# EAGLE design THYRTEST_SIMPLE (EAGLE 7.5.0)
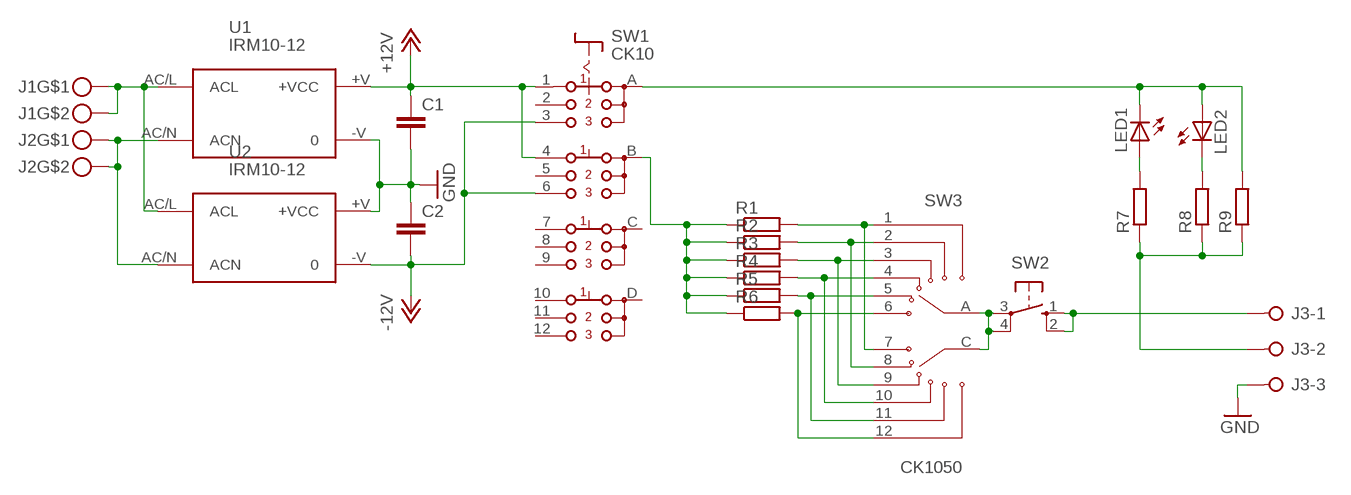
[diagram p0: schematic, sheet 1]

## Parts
C1  C-EUC1206  [C1206]
C2  C-EUC1206  [C1206]
J1  MKDSN1,5-2-5,08  [MKDSN1,5-2-5,08]
J2  MKDSN1,5-2-5,08  [MKDSN1,5-2-5,08]
J3  W237-3E  [W237-3E]
LED1  LED5MM  [LED5MM]
LED2  LED5MM  [LED5MM]
R1  R-EU_M1206  [M1206]
R2  R-EU_M1206  [M1206]
R3  R-EU_M1206  [M1206]
R4  R-EU_M1206  [M1206]
R5  R-EU_M1206  [M1206]
R6  R-EU_M1206  [M1206]
R7  R-EU_M1206  [M1206]
R8  R-EU_M1206  [M1206]
R9  R-EU_R2512  [R2512]
SW1  CK10  [CK10]
SW2  40-XX  [B3F-40XX]
SW3  CK1050  [SW_CK1050]
U1  IRM10-12  [IRM10-12]
U2  IRM10-12  [IRM10-12]

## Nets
+12V: C1.1 SW1.1(A1) SW1.4(B1) U1.+V(+VCC)
-12V: C2.2 SW1.3(A3) SW1.6(B3) U2.-V
GND: C1.2 C2.1 J3.3 U1.-V U2.+V(+VCC)
N$1: J2.1 J2.2 U1.AC/N(ACN) U2.AC/N(ACN)
N$2: R1.1 R2.1 R3.1 R4.1 R5.1 R6.1 SW1.B
N$3: R1.2 SW3.1 SW3.7
N$4: J1.1 J1.2 U1.AC/L(ACL) U2.AC/L(ACL)
N$5: R2.2 SW3.2 SW3.8
N$6: R3.2 SW3.3 SW3.9
N$7: R4.2 SW3.4 SW3.10
N$8: R5.2 SW3.5 SW3.11
N$9: R6.2 SW3.6 SW3.12
N$10: J3.1 SW2.1(S) SW2.2(S1)
N$11: LED1.A R7.2
N$12: LED1.K(C) LED2.A R9.2 SW1.A
N$13: LED2.K(C) R8.2
N$15: SW2.3(P) SW2.4(P1) SW3.A SW3.C
N$17: J3.2 R7.1 R8.1 R9.1
Unconnected: SW1.2(A2) SW1.5(B2) SW1.7(C1) SW1.8(C2) SW1.9(C3) SW1.10(D1) SW1.11(D2) SW1.12(D3) SW1.C SW1.D

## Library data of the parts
C1 C2 = rcl:C-EU: CAPACITOR, European symbol
J1 J2 = con-phoenix-508:MKDSN1,5-2-5,08
J3 = con-wago-508:W237-3E: WAGO SREW CLAMP; OC_FARNELL: unknown; OC_NEWARK: unknown
LED1 LED2 = led:LED: LED
R1-R9 = rcl:R-EU_: RESISTOR, European symbol
SW1 = switch:CK10: ROTARY SWITCH C&K
SW2 = switch-omron:40-XX: OMRON SWITCH; MF: OMRON COMPONENTS USA; MPN: B3F-4000; OC_FARNELL: 176434; OC_NEWARK: 36K3105
SW3 = CK1050:CK1050: Check availability; AVAILABILITY: In Stock; CHECK_PRICES: https://www.snapeda.com/parts/CK1050/Lorlin/view-part/?ref=eda; DESCRIPTION: Rotary wafer switch,metric,BBM,2P 6way | Lorlin CK1050; MF: Lorlin; MP: CK1050; PACKAGE: None; PRICE: None; SNAPEDA_LINK: https://www.snapeda.com/parts/CK1050/Lorlin/view-part/?ref=snap
U1 U2 = acdc:IRM10-12

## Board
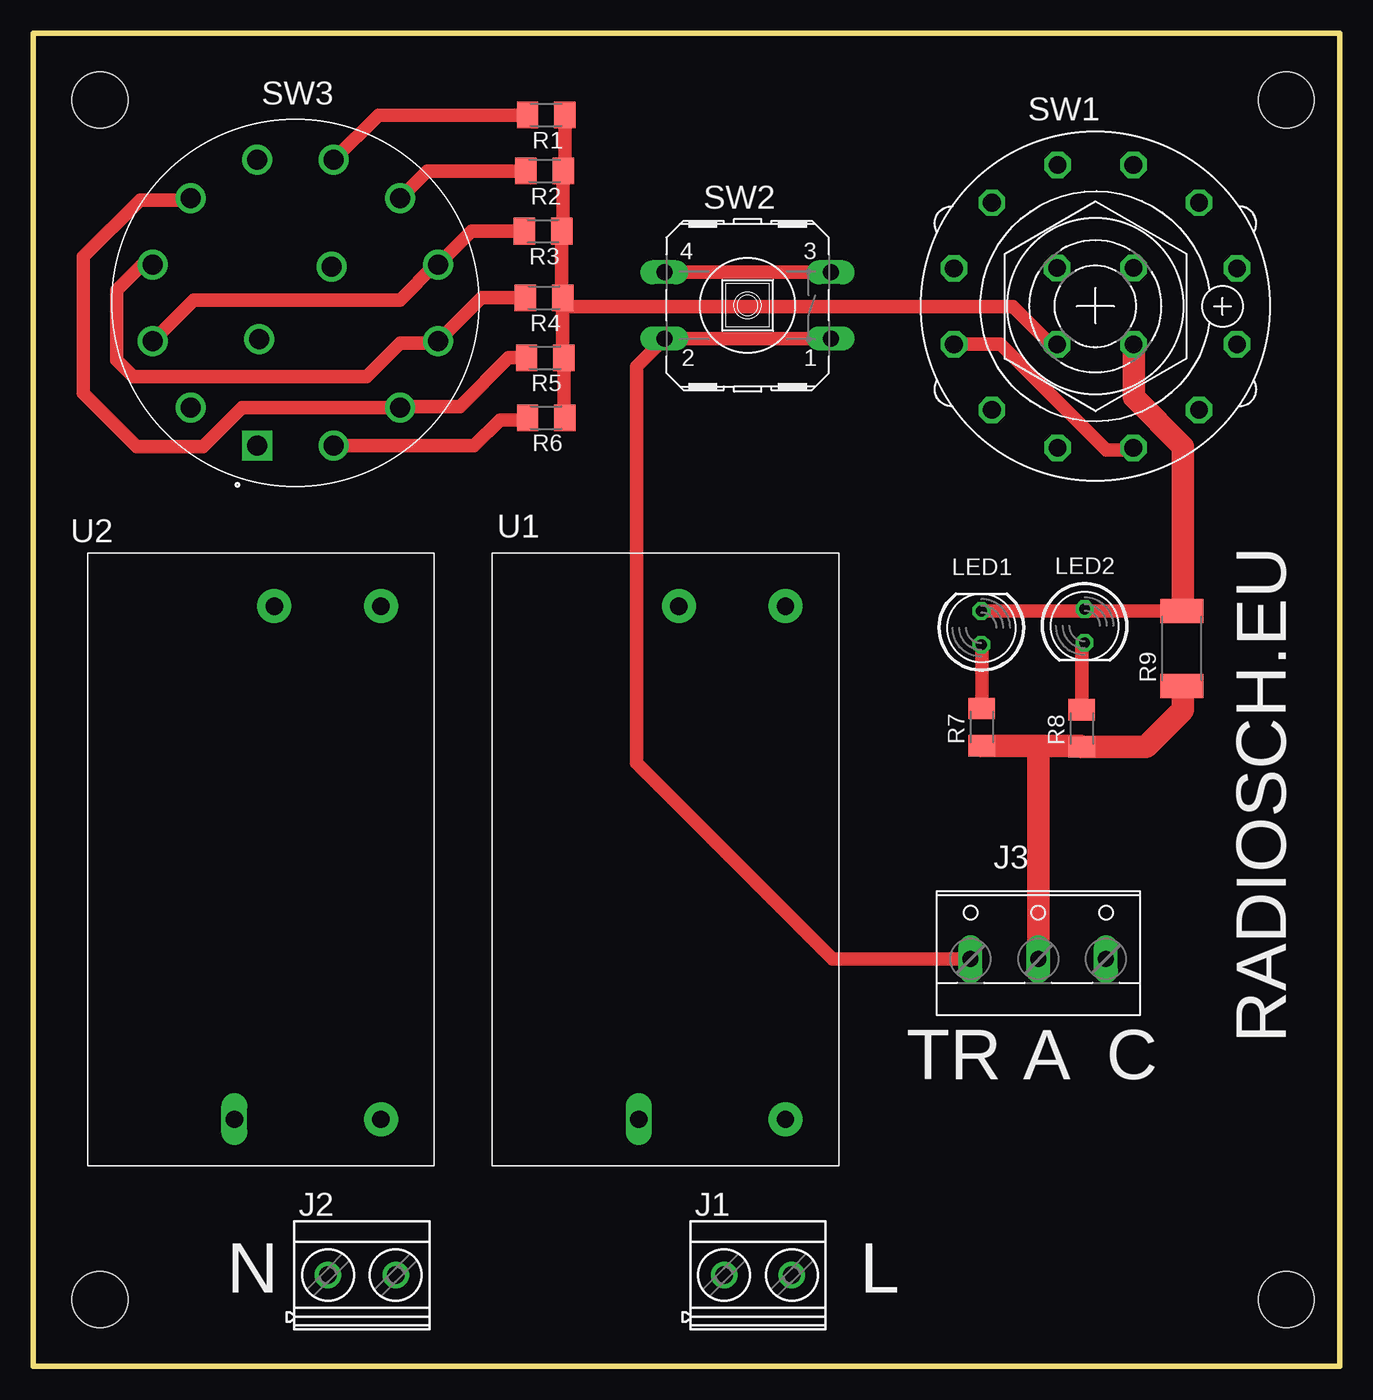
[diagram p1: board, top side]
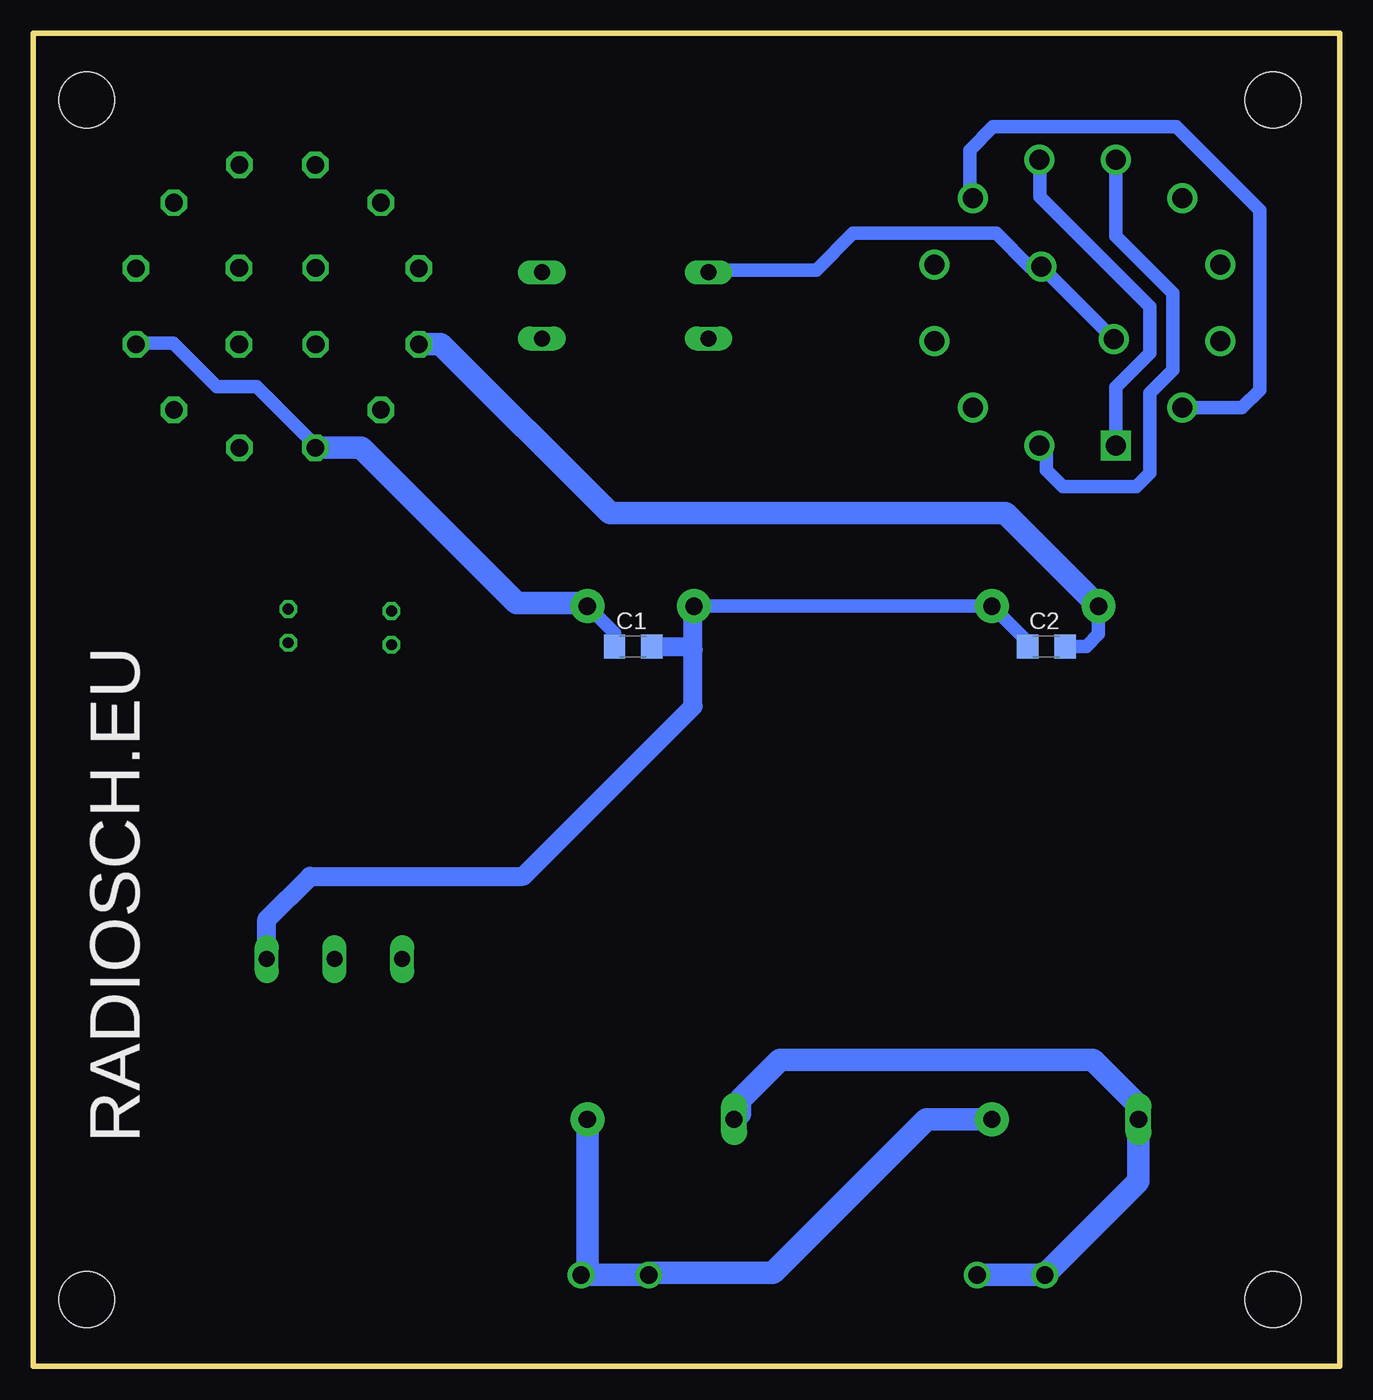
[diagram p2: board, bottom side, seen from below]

Size 98 x 100 mm. Coordinates in mm from the lower left corner, seen from the top.
Outline: 0,0 98,0 98,100 0,100 0,0
Copper layers (1*16): Top 0.035mm / dielectric 1.5mm / Bottom 0.035mm
Design rules "default": minimum track width 10mil, minimum drill 24mil, track to track 8mil, track to pad 8mil, pad to pad 8mil, via to via 8mil, smd to smd 8mil, copper to edge 40mil, drill to drill 8mil, minimum pad ring 10mil, minimum via ring 8mil, stop-mask expansion 4mil, vias tented up to drill 0mil, thermal gap 10mil
Holes 4.2 mm at 5,5 94,5 5,95 94,95

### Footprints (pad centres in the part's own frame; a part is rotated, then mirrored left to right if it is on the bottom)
C1206 = smd 1.6 x 1.8: 1 -1.4,0; 2 1.4,0
MKDSN1,5-2-5,08 = drill 1.3 pad 2: 1 -2.561,0.025; 2 2.519,0.025
W237-3E = drill 1.194 long: 1 -5.08,-0.635; 2 0,-0.635; 3 5.08,-0.635
LED5MM = drill 0.813 octagon: A -1.27,0; K 1.27,0
M1206 = smd 1.6 x 2: 1 -1.4,0; 2 1.4,0
R2512 = smd 1.8 x 3.2: 1 -2.8,0; 2 2.8,0
CK10 = drill 1.321 octagon: 1 -2.845,-10.617; 2 -7.772,-7.772; 3 -10.617,-2.845; 4 -10.617,2.845; 5 -7.772,7.772; 6 -2.845,10.617; 7 2.845,10.617; 8 7.772,7.772; 9 10.617,2.845; 10 10.617,-2.845; 11 7.772,-7.772; 12 2.845,-10.617; A -2.87,-2.87; B -2.87,2.87; C 2.87,2.87; D 2.87,-2.87
B3F-40XX = drill 1.194 long: 1 -6.248,2.489; 2 6.248,2.489; 3 -6.248,-2.489; 4 6.248,-2.489
SW_CK1050 = drill 1.5 square: 1 -2.873,-10.722 | drill 1.5: 2 -7.849,-7.849; 3 -10.722,-2.873; 4 -10.722,2.873; 5 -7.849,7.849; 6 -2.873,10.722; 7 2.873,10.722; 8 7.849,7.849; 9 10.722,2.873; 10 10.722,-2.873; 11 7.849,-7.849; 12 2.873,-10.722; A -2.722,-2.722; C 2.722,2.722
IRM10-12 = drill 1.3 pad 2.54: +V 38.5,0; -V 38.5,8; AC/L 0,0 | drill 1.3 long: AC/N 0,11

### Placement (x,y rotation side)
C1  53,54 0 bottom
C2  22,54 0 bottom
J1  54.39,6.82 0 top
J2  24.67,6.82 0 top
J3  75.4,31.18 0 top
LED1  71.13,55.39 90 top
LED2  78.87,55.54 270 top
R1  38.48,93.87 180 top
R2  38.36,89.67 180 top
R3  38.24,85.16 180 top
R4  38.32,80.16 180 top
R5  38.4,75.66 180 top
R6  38.48,71.16 180 top
R7  71.16,47.94 90 top
R8  78.66,47.86 90 top
R9  86.17,53.84 90 top
SW1  79.69,79.52 90 top
SW2  53.59,79.59 180 top
SW3  19.66,79.78 0 top
U1  56.43,18.52 90 top
U2  26.08,18.52 90 top

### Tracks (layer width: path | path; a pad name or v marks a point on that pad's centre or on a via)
+12V
  Bottom 1.016: SW1.4 76.84,69.09 81.25,73.5 84.25,73.5 87.5,76.75 90.23,76.75 SW1.1 | C1.1 54.4,54.99 U1.+V
  Bottom 1.676: SW1.4 73.4,68.9 61.75,57.25 56.66,57.25 U1.+V
-12V
  Top 1.016: SW1.6 72.58,76.67 80.5,68.75 82.38,68.75 SW1.3
  Bottom 1.016: U2.-V 18.08,54.92 19,54 C2.2
  Bottom 1.676: SW1.6 67.42,76.67 54.75,64 25.06,64 U2.-V
GND
  Bottom 1.016: 48.75,55 48.75,56.7 U1.-V U2.+V 23.4,54.34 C2.1
  Bottom 1.422: J3.3 80.48,33.52 77.25,36.75 61.25,36.75 48.5,49.5 48.5,53.75 | 48.5,53.75 48.5,56.95 U1.-V | C1.2 48.75,54 48.5,53.75
N$1
  Bottom 1.676: U1.AC/N 45,18.95 45,20 42,23 18.5,23 15.08,19.58 U2.AC/N 15.08,13.87 J2.1 J2.2
N$2
  Top 1.016: R1.1 39.88,89.79 R2.1 39.76,85.28 R3.1 39.64,80.24 R4.1 | R4.1 39.72,75.74 R5.1 39.8,71.24 R6.1 | SW1.B 76.35,76.65 73.5,79.5 40.38,79.5 R4.1
N$3
  Top 1.016: R1.2 25.9,93.87 SW3.7
  Bottom 1.016: SW3.1 16.79,73.46 14.25,76 14.25,79.5 22.5,87.75 22.5,90.47 SW3.7
N$4
  Bottom 1.676: U1.AC/L 56.43,7.32 J1.2 J1.1 51.67,7 42.5,7 30.98,18.52 U2.AC/L
N$5
  Top 1.016: R2.2 29.55,89.67 SW3.8
  Bottom 1.016: SW3.2 7.32,71.93 6,73.25 6,86.75 12.25,93 26,93 27.75,91.25 27.75,87.87 SW3.8
N$6
  Top 1.016: R3.2 32.89,85.16 SW3.9 30.15,82.65 27.5,80 12.03,80 SW3.3
N$7
  Top 1.016: R4.2 33.63,80.16 SW3.10 30.23,76.75 27.5,76.75 25,74.25 7.5,74.25 6.25,75.5 6.25,80.75 8.15,82.65 SW3.4
N$8
  Top 1.016: R5.2 35.66,75.66 32,72 27.58,72 SW3.11 15.68,71.93 12.75,69 7.75,69 3.75,73 3.75,83.25 8,87.5 11.68,87.5 SW3.5
N$9
  Top 1.016: SW3.12 33.06,69.06 35,71 36.92,71 R6.2
  Bottom 1.016: SW3.6 16.79,84.79 12.5,80.5 12.5,74.75 14.25,73 14.25,67 15.25,66 20.75,66 22,67.25 22,68.53 SW3.12
N$10
  Top 1.016: J3.1 59.95,30.55 45.25,45.25 45.25,75.01 SW2.2 SW2.1
N$11
  Top 1.016: R7.2 71.16,54.09 LED1.A
N$12
  Top 1.016: R9.2 79.04,56.64 LED2.A 78.72,56.66 LED1.K
  Top 1.676: SW1.A 82.56,72.69 86.25,69 86.25,56.72 R9.2
N$13
  Top 1.016: R8.2 78.66,54.06 LED2.K
N$15
  Top 1.016: SW2.4 SW2.3
  Bottom 1.016: SW3.A SW3.C 23.25,82.5 25.75,85 36.5,85 39.25,82.25 47.17,82.25 SW2.4
N$17
  Top 1.016: 78.58,46.54 R8.1 | 75.4,46.14 75,46.54
  Top 1.676: R7.1 75,46.54 78.58,46.54 | J3.2 75.4,46.14 | R8.1 83.46,46.46 86.25,49.25 86.25,50.96 R9.1

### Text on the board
tPlace: RADIOSCH.EU | TR | A | C | N | L
bPlace: RADIOSCH.EU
